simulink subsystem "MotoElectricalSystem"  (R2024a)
settings: Solver=VariableStepAuto  StartTime=0.0  StopTime=10.0  RelTol=1e-3
undefined symbols (not defined in the file): PlntDCDCVoltInit

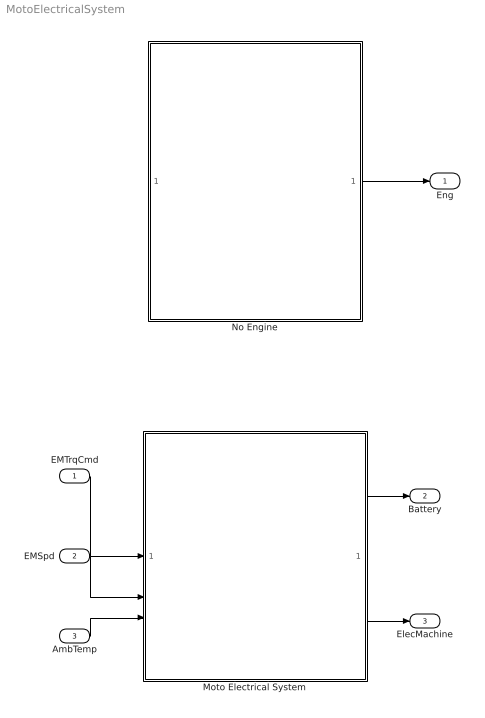
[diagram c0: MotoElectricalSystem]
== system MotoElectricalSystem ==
  EMTrqCmd : Inport
  EMSpd : Inport  Port=2
  AmbTemp : Inport  Port=3
  Moto Electrical System : Subsystem  VariantControl=Moto Electrical System 1EM
  No Engine : Subsystem  VariantControl=No Engine
  Eng : Outport
  Battery : Outport  Port=2
  ElecMachine : Outport  Port=3
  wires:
  AmbTemp/1 -> Moto Electrical System/3(AmbTemp)
  EMSpd/1 -> Moto Electrical System/2(EMSpd)
  EMTrqCmd/1 -> Moto Electrical System/1(EMTrqCmd)
  Moto Electrical System/2(Bus Element Out1) -> ElecMachine/1
  Moto Electrical System/1(Bus Element Out2) -> Battery/1
  No Engine/1(Eng) -> Eng/1

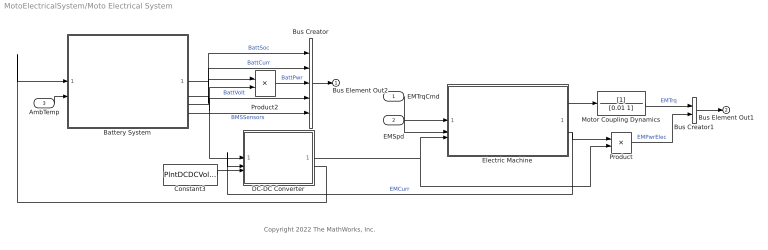
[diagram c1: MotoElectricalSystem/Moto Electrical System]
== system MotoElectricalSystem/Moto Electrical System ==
  note: Copyright 2022 The MathWorks, Inc.
  EMTrqCmd : Inport
  EMSpd : Inport  Port=2
  AmbTemp : Inport  Port=3
  Battery System : Subsystem  Variant=on  VariantControlMode=label  LabelModeActiveChoice=Ideal Voltage Source
  Bus Creator : BusCreator  Inputs=5
  Bus Creator1 : BusCreator  Inputs=2
  Constant3 : Constant  Value=PlntDCDCVoltInit  SampleTime=-1
  DC-DC Converter : Subsystem  Variant=on  VariantControlMode=label  VariantControl=Choice  LabelModeActiveChoice=No DC-DC Converter
  Electric Machine : Subsystem  Variant=on  VariantControlMode=label  LabelModeActiveChoice=Mapped EM
  Motor Coupling Dynamics : TransferFcn  Denominator=[0.01 1]
  Product : Product
  Product2 : Product
  Bus Element Out2 : Outport
  Bus Element Out1 : Outport  Port=2
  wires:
  AmbTemp/1 -> Battery System/2(BattTemp)
  Battery System/2(BattCurr) -> Bus Creator/2, Product2/1  "BattCurr"
  EMTrqCmd/1 -> Electric Machine/1(EMTrqCmd)
  Electric Machine/2(EMCurr) -> DC-DC Converter/2(LdCurr), Product/1  "EMCurr"
  Battery System/1(BattSoc) -> Bus Creator/1  "BattSoc"
  EMSpd/1 -> Electric Machine/2(EMSpd)
  Battery System/3(BattVolt) -> DC-DC Converter/1(BatVolt), Bus Creator/4, Product2/2  "BattVolt"
  Product2/1 -> Bus Creator/3  "BattPwr"
  Product/1 -> Bus Creator1/2  "EMPwrElec"
  Bus Creator1/1 -> Bus Element Out1/1
  Motor Coupling Dynamics/1 -> Bus Creator1/1  "EMTrq"
  Electric Machine/1(EMTrq) -> Motor Coupling Dynamics/1
  Bus Creator/1 -> Bus Element Out2/1
  DC-DC Converter/1(BusVolt) -> Product/2, Electric Machine/3(BusVolt)
  DC-DC Converter/2(SrcCurr) -> Battery System/1(LdCurr)
  Constant3/1 -> DC-DC Converter/3(VoltCmd)
  Battery System/4(BMSSensors) -> Bus Creator/5  "BMSSensors"

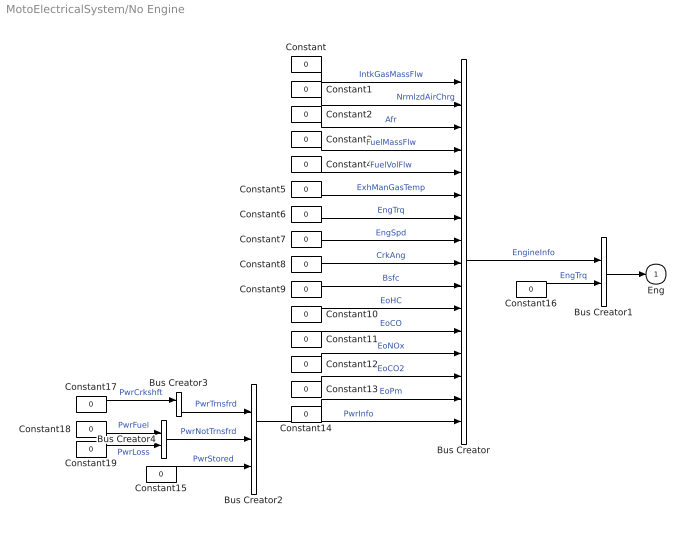
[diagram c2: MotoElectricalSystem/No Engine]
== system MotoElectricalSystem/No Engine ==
  Bus Creator : BusCreator  Inputs=16
  Bus Creator1 : BusCreator  Inputs=2
  Bus Creator2 : BusCreator  Inputs=3
  Bus Creator3 : BusCreator  Inputs=1
  Bus Creator4 : BusCreator  Inputs=2
  Constant{,1..19} (20 alike) : Constant  Value=0
  Eng : Outport
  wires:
  Constant19/1 -> Bus Creator4/2  "PwrLoss"
  Constant18/1 -> Bus Creator4/1  "PwrFuel"
  Constant17/1 -> Bus Creator3/1  "PwrCrkshft"
  Constant15/1 -> Bus Creator2/3  "PwrStored"
  Bus Creator4/1 -> Bus Creator2/2  "PwrNotTrnsfrd"
  Bus Creator3/1 -> Bus Creator2/1  "PwrTrnsfrd"
  Constant16/1 -> Bus Creator1/2  "EngTrq"
  Bus Creator/1 -> Bus Creator1/1  "EngineInfo"
  Bus Creator1/1 -> Eng/1
  Constant5/1 -> Bus Creator/6  "ExhManGasTemp"
  Constant/1 -> Bus Creator/1  "IntkGasMassFlw"
  Constant12/1 -> Bus Creator/13  "EoNOx"
  Constant13/1 -> Bus Creator/14  "EoCO2"
  Bus Creator2/1 -> Bus Creator/16  "PwrInfo"
  Constant3/1 -> Bus Creator/4  "FuelMassFlw"
  Constant1/1 -> Bus Creator/2  "NrmlzdAirChrg"
  Constant14/1 -> Bus Creator/15  "EoPm"
  Constant11/1 -> Bus Creator/12  "EoCO"
  Constant10/1 -> Bus Creator/11  "EoHC"
  Constant8/1 -> Bus Creator/9  "CrkAng"
  Constant7/1 -> Bus Creator/8  "EngSpd"
  Constant4/1 -> Bus Creator/5  "FuelVolFlw"
  Constant6/1 -> Bus Creator/7  "EngTrq"
  Constant2/1 -> Bus Creator/3  "Afr"
  Constant9/1 -> Bus Creator/10  "Bsfc"

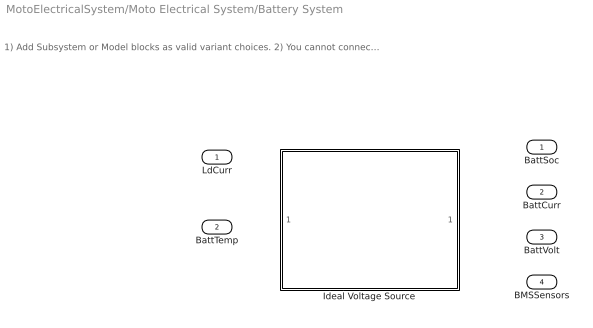
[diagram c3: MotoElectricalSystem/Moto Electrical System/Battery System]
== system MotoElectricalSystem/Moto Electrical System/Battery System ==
  note: 1) Add Subsystem or Model blocks as valid variant choices. 2) You cannot connect blocks at this level. At simulation, connectivity is automatically determined, based on the active variant and port name matching.
  LdCurr : Inport
  BattTemp : Inport  Port=2
  Ideal Voltage Source : Subsystem  VariantControl=Ideal Voltage Source  ReferencedSubsystem=IdealVoltageSource
  BattSoc : Outport  VectorParamsAs1DForOutWhenUnconnected=off
  BattCurr : Outport  Port=2  VectorParamsAs1DForOutWhenUnconnected=off
  BattVolt : Outport  Port=3  VectorParamsAs1DForOutWhenUnconnected=off
  BMSSensors : Outport  Port=4  VectorParamsAs1DForOutWhenUnconnected=off

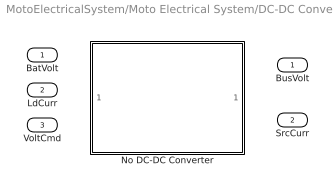
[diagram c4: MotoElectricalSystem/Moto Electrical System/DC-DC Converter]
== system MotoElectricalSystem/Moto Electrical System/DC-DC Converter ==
  BatVolt : Inport
  LdCurr : Inport  Port=2
  VoltCmd : Inport  Port=3
  No DC-DC Converter : Subsystem  VariantControl=No DC-DC Converter  ReferencedSubsystem=NoDCDCConverter
  BusVolt : Outport
  SrcCurr : Outport  Port=2

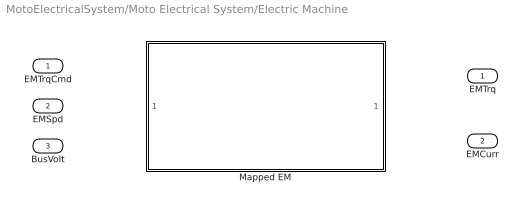
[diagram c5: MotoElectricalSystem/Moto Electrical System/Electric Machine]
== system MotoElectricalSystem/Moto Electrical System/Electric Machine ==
  EMTrqCmd : Inport
  EMSpd : Inport  Port=2
  BusVolt : Inport  Port=3
  Mapped EM : Subsystem  VariantControl=Mapped EM  ReferencedSubsystem=ElectricMachine1
  EMTrq : Outport  VectorParamsAs1DForOutWhenUnconnected=off
  EMCurr : Outport  Port=2  VectorParamsAs1DForOutWhenUnconnected=off
